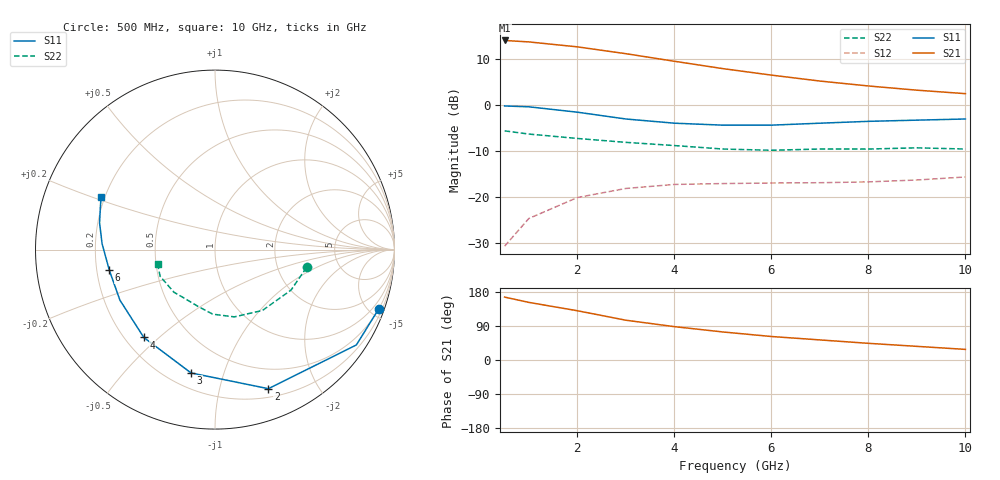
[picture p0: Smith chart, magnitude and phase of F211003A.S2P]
!ATF-21100
!S-PARAMETERS at Vds=3V  Id=20mA.  LAST UPDATED 07-22-92
# ghz s ma r 50
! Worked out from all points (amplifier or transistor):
!   11 points, 500 MHz to 10 GHz, reference 50 ohm
!   highest |S21| = 14.0 dB at 500 MHz (marker M1)
!   |S21| within 3 dB of that: start of sweep to 3.074 GHz
!   unconditionally stable (mu >= 1): 6.714 GHz to end of sweep
!   at 1 GHz: K = 0.14, MSG = 19.2 dB, |S12| = -24.7 dB
!   at 5 GHz: K = 0.81, MSG = 12.5 dB, |S12| = -17.1 dB
!   at 10 GHz: K = 1.06, MAG = 7.5 dB, |S12| = -15.7 dB
!   lowest NFmin = 0.50 dB at 100 MHz
!   S11 on the Smith chart (normalised r, x): 500 MHz: 0.50, -5.63; 2 GHz: 0.28, -1.42; 3 GHz: 0.29, -0.78; 4 GHz: 0.28, -0.45; 6 GHz: 0.25, -0.09; 10 GHz: 0.18, +0.21
0.5  0.97 -20.0  5 166.0  0.029 77.0  0.52 -11.0
1  0.95 -34.0  4.82 152.0  0.058 73.0  0.48 -28.0
2  0.83 -69.0  4.26 130.0  0.098 56.0  0.43 -52.0
3  0.7 -101.0  3.59 105.0  0.123 45.0  0.39 -74.0
4  0.63 -129.0  2.97 88.0  0.136 39.0  0.36 -92.0
5  0.6 -152.0  2.47 74.0  0.139 36.0  0.33 -107.0
6  0.6 -169.0  2.1 62.0  0.141 34.0  0.32 -122.0
7  0.63 177.0  1.81 53.0  0.142 33.0  0.33 -134.0
8  0.66 167.0  1.6 44.0  0.145 32.0  0.33 -145.0
9  0.68 160.0  1.44 36.0  0.152 31.0  0.34 -154.0
10  0.7 155.0  1.32 28.0  0.164 27.0  0.33 -166.0
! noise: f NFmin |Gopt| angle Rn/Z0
0.1  0.5  0.99  1  1
2  0.6  0.72  42  0.64
4  0.9  0.61  104  0.28
6  1.2  0.55  160  0.07
